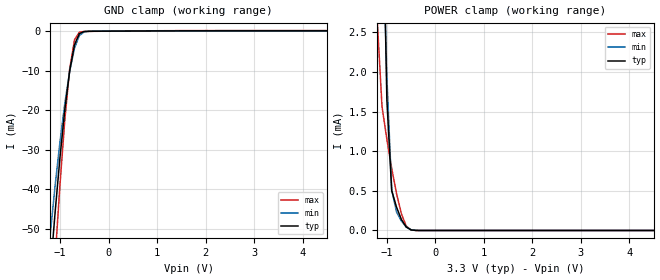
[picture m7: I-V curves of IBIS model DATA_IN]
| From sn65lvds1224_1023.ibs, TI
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|   Model DATA_IN
|Developed by Ayah el_khordagy
[Model]   DATA_IN
Model_type   Input
Polarity   Non-Inverting
| Vinl and Vinh from datasheet.
Vinl = 0.8
Vinh = 2.0
| C_comp values are extracted by ICX.
C_comp   1.26pF   1.14pF   1.39pF
[Temperature Range]   27   85   -40
[Voltage Range]   3.3V   3.0V   3.6V
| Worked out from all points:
|   GND clamp passes 1 mA (typ) near -0.61 V on its own axis
|   POWER clamp passes 1 mA (typ) near -0.94 V on its own axis
[GND_clamp]
| voltage   I(typ)   I(min)   I(max)
-3.3V     -472.1mA   -392.6mA   -586.9mA
-1.2V     -60.92mA   -51.25mA   -77.93mA
-1.1V     -45.73mA   -39.03mA   -57.5mA
-1V       -31.91mA   -27.97mA   -38.75mA
-900mV    -19.83mA   -18.24mA   -22.37mA
-800mV    -10.04mA   -10.15mA   -9.541mA
-700mV    -3.419mA   -4.259mA   -2.163mA
-600mV    -613.9uA   -1.115mA   -246.7uA
-500mV    -88.05uA   -185uA     -74.65uA
-300mV    -22.88uA   -16.8uA    -40.47uA
6.6V      80.26uA    50.2uA     150.8uA
[POWER_clamp]
| voltage   I(typ)   I(min)   I(max)
-3.3V     119.6mA    83.59mA    139.9mA
-1.2V     8.578mA    6.685mA    2.677mA
-1.1V     4.813mA    4.138mA    1.562mA
-1V       1.65mA     1.939mA    1.151mA
-900mV    501.8uA    512.5uA    783.1uA
-800mV    292.8uA    232.5uA    463uA
-700mV    138.4uA    118.4uA    210uA
-600mV    42.94uA    43.54uA    55.3uA
-500mV    6.94uA     9.34uA     6.6uA
-300mV    50nA       100nA      100nA
6.6V      0A         0A         0A
